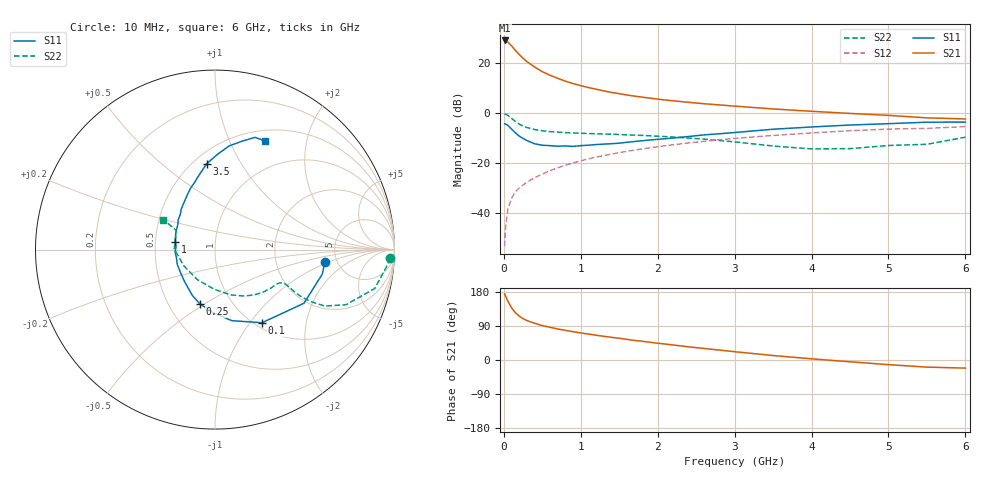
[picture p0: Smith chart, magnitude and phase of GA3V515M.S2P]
! Infineon Technologies  Discrete & RF Semiconductors
! BF775
! Si NPN RF Bipolar Junction Transistor in SOT23
! VCE = 3.5 V  IC = 15 mA
! Common Emitter S-Parameters:  May  1996
# GHz  S  MA  R  50
!  f  S11  S21  S12  S22
! GHz  MAG  ANG  MAG  ANG  MAG  ANG  MAG  ANG
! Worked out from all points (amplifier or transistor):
!   36 points, 10 MHz to 6 GHz, reference 50 ohm
!   highest |S21| = 29.1 dB at 10 MHz (marker M1)
!   |S21| within 3 dB of that: start of sweep to 122.8 MHz
!   unconditionally stable (mu >= 1): 454.1 MHz to 3.119 GHz
!   at 250 MHz: K = 0.80, MSG = 25.3 dB, |S12| = -28.7 dB
!   at 1.4 GHz: K = 1.11, MAG = 10.3 dB, |S12| = -16.3 dB
!   at 6 GHz: K = 0.95, MSG = 1.5 dB, |S12| = -5.3 dB
!   S11 on the Smith chart (normalised r, x): 10 MHz: 3.99, -0.90; 100 MHz: 1.08, -1.15; 250 MHz: 0.71, -0.48; 1 GHz: 0.64, +0.06; 3.5 GHz: 0.58, +0.72; 6 GHz: 0.63, +1.36
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0.01  0.6157 -6.5  28.64 174.7  0.0022 86.0  0.9759 -2.8
0.02  0.6132 -12.9  28.15 169.7  0.0047 80.0  0.9606 -5.7
0.05  0.5787 -31.1  26.66 156.1  0.0117 78.5  0.9157 -13.7
0.1  0.4846 -57.2  22.31 137.9  0.02 69.5  0.7921 -22.8
0.15  0.407 -76.7  18.08 124.5  0.0269 65.5  0.6878 -27.2
0.2  0.3497 -92.4  14.99 115.7  0.0321 64.8  0.6093 -28.5
0.25  0.3134 -105.6  12.57 109.1  0.0368 64.8  0.555 -28.7
0.3  0.285 -116.3  10.81 104.1  0.042 65.0  0.519 -28.3
0.4  0.2456 -134.0  8.417 96.9  0.0514 66.4  0.474 -27.2
0.5  0.2297 -148.2  6.814 90.9  0.0609 67.5  0.4461 -26.3
0.6  0.2254 -158.9  5.773 86.3  0.0714 67.7  0.4304 -26.0
0.7  0.2196 -168.5  5.005 81.9  0.0811 68.4  0.4204 -26.4
0.8  0.2228 -176.6  4.392 78.2  0.0915 67.7  0.4108 -26.8
1  0.2255 168.7  3.574 71.4  0.1122 67.3  0.3997 -28.2
1.1  0.2299 162.9  3.274 68.5  0.1226 66.6  0.3933 -29.4
1.3  0.2419 152.5  2.8 62.5  0.143 64.9  0.3848 -32.0
1.6  0.263 141.5  2.322 54.4  0.1738 62.3  0.3704 -36.7
2.2  0.3201 121.8  1.776 39.6  0.2349 55.9  0.3358 -48.4
3.5  0.4802 95.6  1.222 11.8  0.3604 39.7  0.2215 -91.0
4.5  0.5829 82.2  0.994 -4.7  0.4481 26.4  0.1964 -153.1
5.5  0.664 70.4  0.81 -18.8  0.4985 11.6  0.24 153.8
6  0.6657 65.3  0.771 -21.4  0.543 7.5  0.3327 149.8
